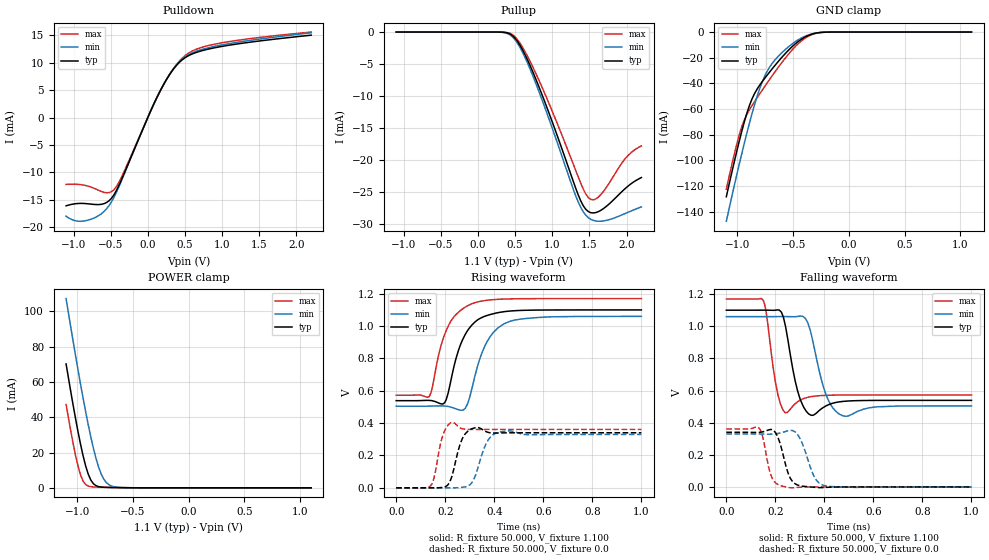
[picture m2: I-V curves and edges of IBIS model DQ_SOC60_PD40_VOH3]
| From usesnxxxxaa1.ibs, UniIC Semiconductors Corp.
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|   Model DQ_SOC60_PD40_VOH3
[Model] DQ_SOC60_PD40_VOH3
Model_type I/O
Polarity   Non-Inverting
Enable   Active-High
Vinl =  0.113V
Vinh =  0.253V
Vmeas =  0.183V
Rref =  50.000
Vref =  0.183V
C_comp   1.110pF   1.087pF   1.118pF
[Model Spec]
Vinh   0.253V   0.247V   0.265V
Vinl   0.113V   0.107V   0.125V
Vmeas   0.183V   NA   NA
Vref   0.183V   NA   NA
Rref   50.000   NA   NA
[Temperature Range]   25.000   0.125k   -40.000
[Voltage Range]   1.100V   1.060V   1.170V
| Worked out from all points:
|   slope of the pulldown table from 0 to 0.165 V, typ, clamps not added: 34.3 ohm
|   GND clamp passes 1 mA (typ) near -0.30 V on its own axis
|   POWER clamp passes 1 mA (typ) near -0.82 V on its own axis
|   rising waveform, R_fixture 50.000, V_fixture 1.100: 20-80 % time 77.2ps typ, 81.2ps min, 75.9ps max; typ from 0.539 V to 1.1 V
|   rising waveform, R_fixture 50.000, V_fixture 0.0: 20-80 % time 34.7ps typ, 43.7ps min, 27.8ps max; typ from 0 V to 0.34 V
|   falling waveform, R_fixture 50.000, V_fixture 1.100: 20-80 % time 39.3ps typ, 50.8ps min, 30.3ps max; typ from 1.1 V to 0.539 V
|   falling waveform, R_fixture 50.000, V_fixture 0.0: 20-80 % time 38ps typ, 46.2ps min, 30.4ps max; typ from 0.34 V to 0 V
[Pulldown]
|Voltage   I(typ)   I(min)   I(max)
-1.1V     -16.12mA   -18.01mA   -12.21mA
-930mV    -15.69mA   -18.94mA   -12.21mA
-726mV    -15.86mA   -18.36mA   -12.9mA
-556mV    -15.52mA   -16.68mA   -13.74mA
-454mV    -14.08mA   -14.53mA   -13.16mA
-352mV    -11.27mA   -11.46mA   -10.83mA
158mV     4.629mA    4.648mA    4.586mA
328mV     8.522mA    8.602mA    8.586mA
498mV     10.89mA    11.05mA    11.26mA
668mV     11.95mA    12.17mA    12.54mA
940mV     12.84mA    13.11mA    13.5mA
2.2V      15.04mA    15.47mA    15.61mA
[Pullup]
|Voltage   I(typ)   I(min)   I(max)
-1.1V     1nA        30.41nA    -1.059nA
432mV     -297.3uA   -442.9uA   -201.3uA
568mV     -2.094mA   -2.448mA   -1.778mA
738mV     -6.208mA   -6.823mA   -5.447mA
976mV     -13.28mA   -14.24mA   -11.72mA
1.316V    -24.43mA   -25.63mA   -21.65mA
1.418V    -27.19mA   -28.13mA   -24.57mA
1.486V    -28.09mA   -29.04mA   -25.91mA
1.554V    -28.31mA   -29.48mA   -26.26mA
1.622V    -28.1mA    -29.61mA   -25.82mA
1.996V    -24.35mA   -28.33mA   -19.63mA
2.2V      -22.77mA   -27.36mA   -17.82mA
[GND_clamp]
|Voltage   I(typ)   I(min)   I(max)
-1.1V     -128.5mA   -147.6mA   -122.6mA
-1.008V   -93.62mA   -112mA     -87.95mA
-962mV    -77.6mA    -95.05mA   -73.96mA
-893mV    -57.36mA   -71.21mA   -60.7mA
-847mV    -48.01mA   -56.81mA   -54.36mA
-801mV    -41.47mA   -44.23mA   -48.33mA
-755mV    -36.02mA   -34.19mA   -42.41mA
-709mV    -30.9mA    -26.94mA   -36.63mA
-525mV    -12.67mA   -10.3mA    -15.49mA
-387mV    -3.615mA   -3.065mA   -4.419mA
-249mV    -281uA     -330.6uA   -301.3uA
1.1V      0A         0A         0A
[POWER_clamp]
|Voltage   I(typ)   I(min)   I(max)
-1.1V     70.27mA    107.3mA    47.25mA
-1.039V   47.68mA    83.93mA    25.86mA
-993mV    31.88mA    66.94mA    12.35mA
-970mV    24.65mA    58.72mA    7.262mA
-947mV    18.06mA    50.74mA    3.761mA
-901mV    7.73mA     35.71mA    987.1uA
-855mV    2.348mA    22.46mA    514uA
-809mV    697.3uA    11.94mA    396.5uA
-763mV    321uA      5.097mA    322.7uA
-717mV    213.8uA    1.813mA    258.1uA
-556mV    65.24uA    79.15uA    81.64uA
1.1V      0A         0A         0A
[Ramp]
| variable   typ   min   max
dV/dt_r   0.204/35.354p   0.198/44.036p   0.217/27.986p
dV/dt_f   0.337/39.679p   0.333/51.882p   0.359/30.346p
R_load = 50.000
[Rising Waveform]
R_fixture= 50.000
V_fixture= 1.100
V_fixture_min= 1.060
V_fixture_max= 1.170
|time   V(typ)   V(min)   V(max)
0s        538.9mV    504.5mV    572.5mV
136ps     540.4mV    505mV      567.5mV
197ps     525.2mV    505.9mV    945.7mV
273ps     922.8mV    481.1mV    1.109V
292ps     974.2mV    522.4mV    1.126V
310ps     1.009V     621.2mV    1.139V
340ps     1.046V     793.2mV    1.152V
374ps     1.067V     912.8mV    1.16V
463ps     1.093V     1.029V     1.168V
1ns       1.1V       1.06V      1.17V
[Rising Waveform]
R_fixture= 50.000
V_fixture= 0.0
V_fixture_min= 0.0
V_fixture_max= 0.0
|time   V(typ)   V(min)   V(max)
0s        1.764uV    14.27uV    330.5nV
140ps     77.8uV     -21.91uV   11.81mV
154ps     -38.97uV   12.68uV    60.13mV
187ps     2.558mV    35uV       308.9mV
223ps     53.97mV    -77.17uV   403.5mV
269ps     301.9mV    3.368mV    365.7mV
323ps     371.8mV    74.98mV    361.1mV
366ps     347.8mV    271.1mV    361.1mV
417ps     339.1mV    343.3mV    361.1mV
1ns       340.3mV    329.8mV    361.1mV
[Falling Waveform]
R_fixture= 50.000
V_fixture= 1.100
V_fixture_min= 1.060
V_fixture_max= 1.170
|time   V(typ)   V(min)   V(max)
0s        1.1V       1.06V      1.17V
151ps     1.1V       1.06V      1.16V
203ps     1.101V     1.06V      629.7mV
240ps     1.009V     1.06V      462.1mV
290ps     601.6mV    1.061V     529.1mV
322ps     480.3mV    1.05V      553.5mV
347ps     445.5mV    946.3mV    562.3mV
407ps     504.7mV    572.7mV    570.1mV
476ps     532.3mV    442.5mV    572mV
1ns       538.8mV    504.5mV    572.5mV
[Falling Waveform]
R_fixture= 50.000
V_fixture= 0.0
V_fixture_min= 0.0
V_fixture_max= 0.0
|time   V(typ)   V(min)   V(max)
0s        340.3mV    329.8mV    361.1mV
132ps     339.3mV    329.3mV    369.1mV
146ps     342mV      328.9mV    326.3mV
187ps     355.7mV    328.7mV    54.11mV
213ps     297.9mV    333.2mV    13.26mV
243ps     130.2mV    345.8mV    -235.6uV
292ps     11.04mV    323mV      -2.728mV
357ps     -2.061mV   68.01mV    -138.5uV
397ps     -3.923mV   9.715mV    -16.11uV
1ns       2.588uV    17.55uV    -131.1nV
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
